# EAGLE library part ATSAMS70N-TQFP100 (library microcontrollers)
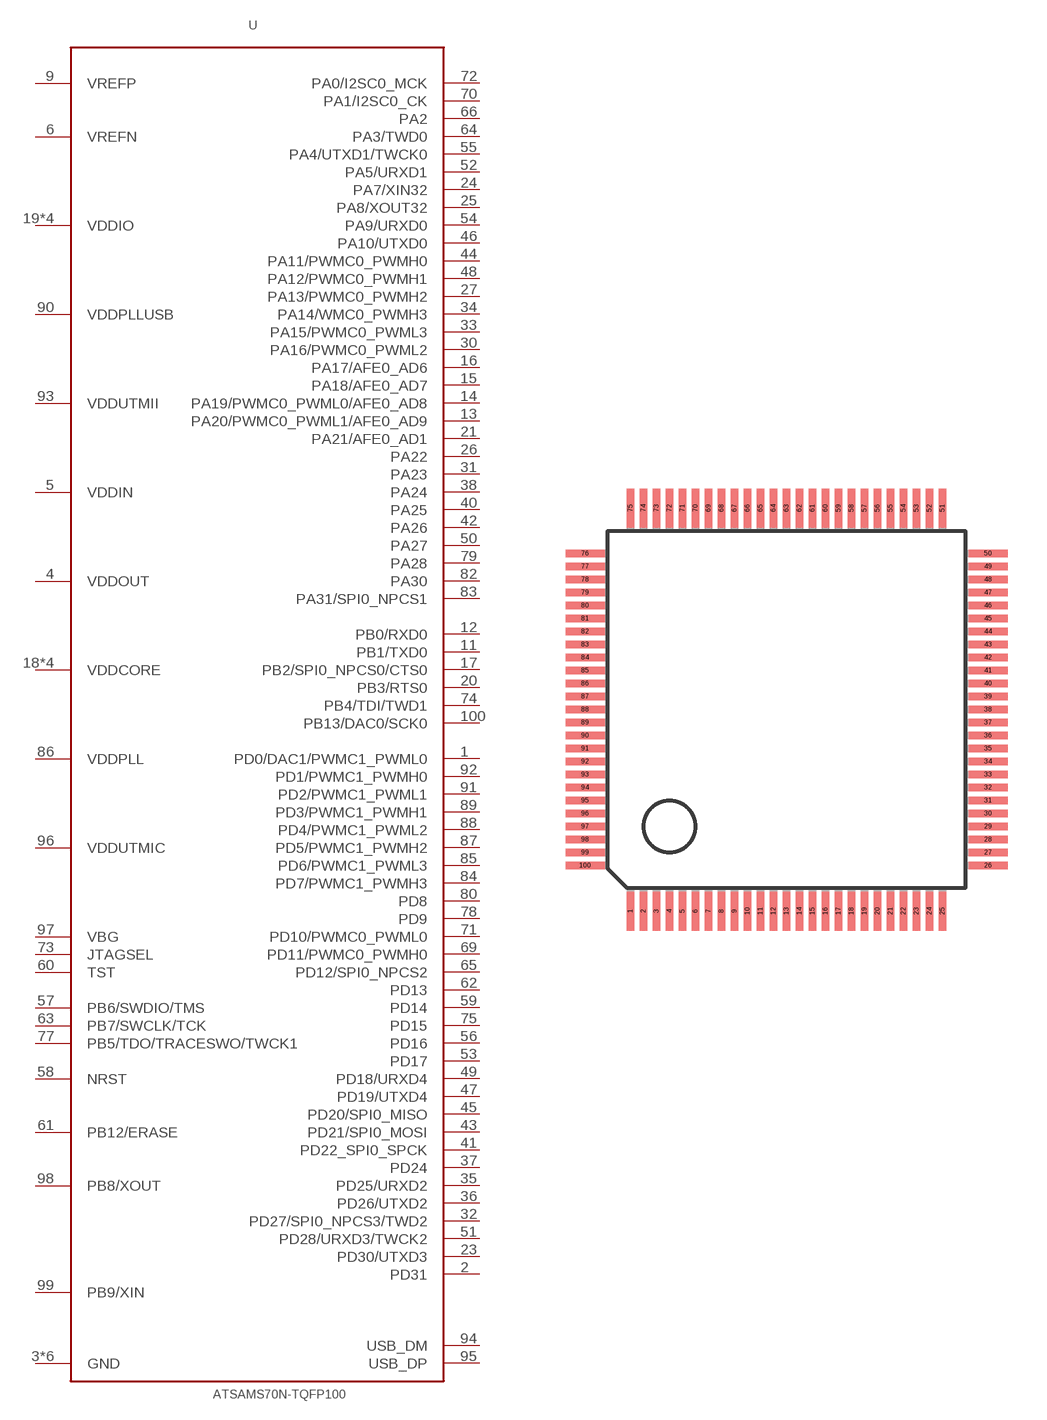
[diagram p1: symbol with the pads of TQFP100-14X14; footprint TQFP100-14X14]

Designator prefix U

## ATSAMS70N-TQFP100  [TQFP100-14X14]
1  PD0/DAC1/PWMC1_PWML0
2  PD31
3  GND
4  VDDOUT
5  VDDIN
6  VREFN
7  GND
8  GND
9  VREFP
10  GND
11  PB1/TXD0
12  PB0/RXD0
13  PA20/PWMC0_PWML1/AFE0_AD9
14  PA19/PWMC0_PWML0/AFE0_AD8
15  PA18/AFE0_AD7
16  PA17/AFE0_AD6
17  PB2/SPI0_NPCS0/CTS0
18  VDDCORE
19  VDDIO
20  PB3/RTS0
21  PA21/AFE0_AD1
22  VDDCORE
23  PD30/UTXD3
24  PA7/XIN32
25  PA8/XOUT32
26  PA22
27  PA13/PWMC0_PWMH2
28  VDDIO
29  GND
30  PA16/PWMC0_PWML2
31  PA23
32  PD27/SPI0_NPCS3/TWD2
33  PA15/PWMC0_PWML3
34  PA14/WMC0_PWMH3
35  PD25/URXD2
36  PD26/UTXD2
37  PD24
38  PA24
39  VDDCORE
40  PA25
41  PD22_SPI0_SPCK
42  PA26
43  PD21/SPI0_MOSI
44  PA11/PWMC0_PWMH0
45  PD20/SPI0_MISO
46  PA10/UTXD0
47  PD19/UTXD4
48  PA12/PWMC0_PWMH1
49  PD18/URXD4
50  PA27
51  PD28/URXD3/TWCK2
52  PA5/URXD1
53  PD17
54  PA9/URXD0
55  PA4/UTXD1/TWCK0
56  PD16
57  PB6/SWDIO/TMS
58  NRST
59  PD14
60  TST
61  PB12/ERASE
62  PD13
63  PB7/SWCLK/TCK
64  PA3/TWD0
65  PD12/SPI0_NPCS2
66  PA2
67  GND
68  VDDIO
69  PD11/PWMC0_PWMH0
70  PA1/I2SC0_CK
71  PD10/PWMC0_PWML0
72  PA0/I2SC0_MCK
73  JTAGSEL
74  PB4/TDI/TWD1
75  PD15
76  VDDCORE
77  PB5/TDO/TRACESWO/TWCK1
78  PD9
79  PA28
80  PD8
81  VDDIO
82  PA30
83  PA31/SPI0_NPCS1
84  PD7/PWMC1_PWMH3
85  PD6/PWMC1_PWML3
86  VDDPLL
87  PD5/PWMC1_PWMH2
88  PD4/PWMC1_PWML2
89  PD3/PWMC1_PWMH1
90  VDDPLLUSB
91  PD2/PWMC1_PWML1
92  PD1/PWMC1_PWMH0
93  VDDUTMII
94  USB_DM
95  USB_DP
96  VDDUTMIC
97  VBG
98  PB8/XOUT
99  PB9/XIN
100  PB13/DAC0/SCK0

## Footprint TQFP100-14X14 (pad centres in mm)
Thin Quad Flat Pack 14x14 mm
smd 0.27 x 1.5: 1 -6,-7.75; 2 -5.5,-7.75; 3 -5,-7.75; 4 -4.5,-7.75; 5 -4,-7.75; 6 -3.5,-7.75; 7 -3,-7.75; 8 -2.5,-7.75; 9 -2,-7.75; 10 -1.5,-7.75; 11 -1,-7.75; 12 -0.5,-7.75; 13 0,-7.75; 14 0.5,-7.75; 15 1,-7.75; 16 1.5,-7.75; 17 2,-7.75; 18 2.5,-7.75; 19 3,-7.75; 20 3.5,-7.75; 21 4,-7.75; 22 4.5,-7.75; 23 5,-7.75; 24 5.5,-7.75; 25 6,-7.75; 51 6,7.75; 52 5.5,7.75; 53 5,7.75; 54 4.5,7.75; 55 4,7.75; 56 3.5,7.75; 57 3,7.75; 58 2.5,7.75; 59 2,7.75; 60 1.5,7.75; 61 1,7.75; 62 0.5,7.75; 63 0,7.75; 64 -0.5,7.75; 65 -1,7.75; 66 -1.5,7.75; 67 -2,7.75; 68 -2.5,7.75; 69 -3,7.75; 70 -3.5,7.75; 71 -4,7.75; 72 -4.5,7.75; 73 -5,7.75; 74 -5.5,7.75; 75 -6,7.75
smd 1.5 x 0.27: 26 7.75,-6; 27 7.75,-5.5; 28 7.75,-5; 29 7.75,-4.5; 30 7.75,-4; 31 7.75,-3.5; 32 7.75,-3; 33 7.75,-2.5; 34 7.75,-2; 35 7.75,-1.5; 36 7.75,-1; 37 7.75,-0.5; 38 7.75,0; 39 7.75,0.5; 40 7.75,1; 41 7.75,1.5; 42 7.75,2; 43 7.75,2.5; 44 7.75,3; 45 7.75,3.5; 46 7.75,4; 47 7.75,4.5; 48 7.75,5; 49 7.75,5.5; 50 7.75,6; 76 -7.75,6; 77 -7.75,5.5; 78 -7.75,5; 79 -7.75,4.5; 80 -7.75,4; 81 -7.75,3.5; 82 -7.75,3; 83 -7.75,2.5; 84 -7.75,2; 85 -7.75,1.5; 86 -7.75,1; 87 -7.75,0.5; 88 -7.75,0; 89 -7.75,-0.5; 90 -7.75,-1; 91 -7.75,-1.5; 92 -7.75,-2; 93 -7.75,-2.5; 94 -7.75,-3; 95 -7.75,-3.5; 96 -7.75,-4; 97 -7.75,-4.5; 98 -7.75,-5; 99 -7.75,-5.5; 100 -7.75,-6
